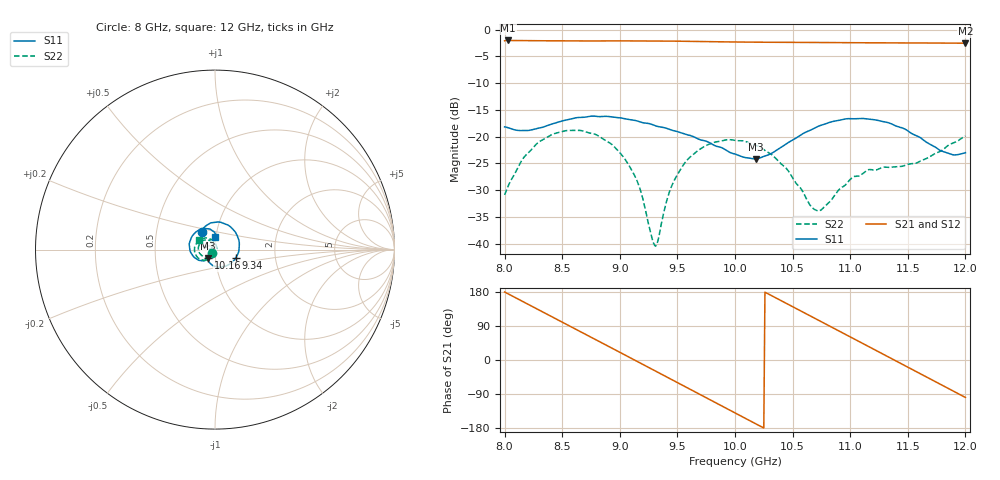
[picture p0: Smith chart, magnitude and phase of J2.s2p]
!Keysight Technologies,N5234A,MY52241180,A.10.60.03
!Date: Tuesday, May 30, 2023 15:17:26
!Correction: S11(Full 2 Port(1,2))
!S21(Full 2 Port(1,2))
!S12(Full 2 Port(1,2))
!S22(Full 2 Port(1,2))
!S2P File: Measurements: S11, S21, S12, S22:
# Hz S  dB  R 50
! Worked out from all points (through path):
!   401 points, 8 GHz to 12 GHz, reference 50 ohm
!   highest |S21| = -2.03 dB at 8.03 GHz (marker M1); lowest = -2.5 dB at 12 GHz (marker M2)
!   group delay of S21, straight-line fit = 443 ps
!   lowest |S11| = -24.2 dB at 10.18 GHz (marker M3), VSWR 1.13, Z = 46.1 - j4.54 ohm
!   |S11| at or under -10 dB: start of sweep to end of sweep
!   |S22| runs from -40.5 to -18.8 dB; largest |S21 - S12| = 0.0015
!   S11 on the Smith chart (normalised r, x): 8 GHz: 0.85, +0.17; 9.34 GHz: 1.25, -0.12; 10.16 GHz: 0.92, -0.09; 12 GHz: 0.98, +0.14
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8e9  -18.18 126.7  -2.09 179.4  -2.09 179.4  -30.89 -132.9
8.03e9  -18.34 126.6  -2.03 174.7  -2.04 174.7  -29.28 -126.1
8.17e9  -18.88 127.7  -2.05 152.3  -2.06 152.3  -23.82 -125.5
8.38e9  -17.86 122.9  -2.09 118.9  -2.10 118.9  -19.98 -148.8
8.67e9  -16.41 93.3  -2.12 72.9  -2.13 72.9  -18.90 169.8
9.02e9  -16.56 38.3  -2.11 17.1  -2.12 17.1  -23.51 116.1
9.16e9  -17.14 12.6  -2.10 -5.4  -2.11 -5.3  -28.83 88.5
9.29e9  -17.82 -12.5  -2.12 -26.2  -2.13 -26.2  -39.78 17.0
9.34e9  -18.16 -22.4  -2.13 -34.3  -2.13 -34.3  -38.64 -60.0
9.44e9  -18.72 -41.7  -2.14 -50.4  -2.15 -50.4  -29.82 -102.1
9.57e9  -19.57 -66.3  -2.18 -71.2  -2.19 -71.2  -24.77 -129.8
9.78e9  -21.15 -100.9  -2.25 -104.8  -2.26 -104.8  -21.39 -162.6
1e10  -23.25 -124.0  -2.31 -139.8  -2.32 -139.8  -20.71 165.8
1.016e10  -24.15 -127.9  -2.35 -165.2  -2.36 -165.2  -21.52 145.6
1.018e10  -24.17 -127.6  -2.35 -168.3  -2.36 -168.3  -21.64 143.3
1.041e10  -21.87 -131.7  -2.38 155.1  -2.39 155.1  -25.27 119.5
1.067e10  -18.64 -154.4  -2.40 113.7  -2.42 113.7  -33.30 132.0
1.098e10  -16.65 166.4  -2.44 64.2  -2.45 64.2  -28.52 176.9
1.134e10  -17.47 119.1  -2.48 6.8  -2.49 6.8  -25.73 163.0
1.152e10  -19.23 99.5  -2.49 -21.9  -2.50 -22.0  -25.10 161.5
1.171e10  -21.62 87.2  -2.50 -52.3  -2.52 -52.4  -23.49 163.7
1.2e10  -23.01 92.2  -2.54 -98.8  -2.55 -98.8  -19.89 149.0
